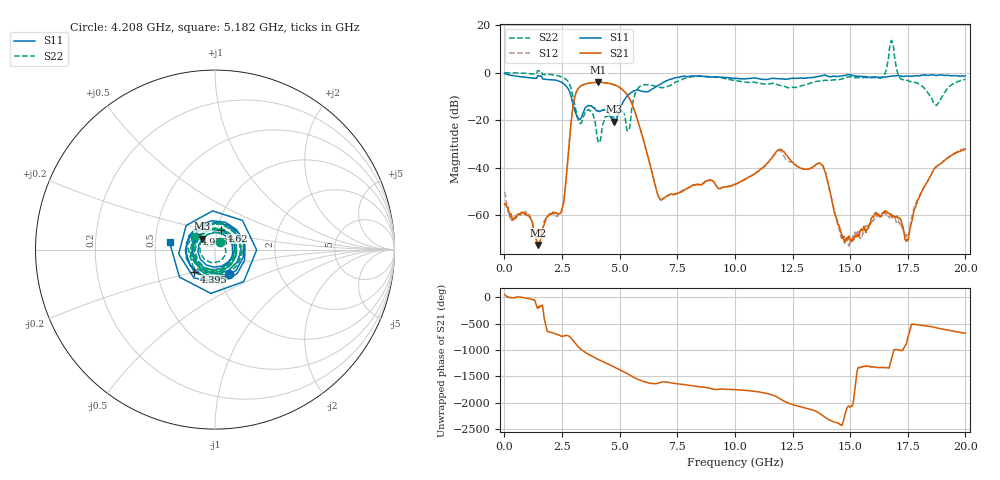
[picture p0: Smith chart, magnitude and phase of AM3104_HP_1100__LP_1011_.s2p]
!Created with skrf (http://scikit-rf.org).
# Hz S RI R 50.0
!freq ReS11 ImS11 ReS21 ImS21 ReS12 ImS12 ReS22 ImS22
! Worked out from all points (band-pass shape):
!   1601 points, 10 MHz to 20 GHz, reference 50 ohm
!   highest |S21| = -4.02 dB at 4.083 GHz (marker M1); lowest = -72.6 dB at 1.459 GHz (marker M2)
!   |S21| within 3 dB of the highest: 3.185 GHz to 5.109 GHz (1.924 GHz wide, 46.4 % of centre)
!   lowest |S11| = -20.6 dB at 4.77 GHz (marker M3), VSWR 1.21, Z = 43.1 + j5.27 ohm
!   |S11| at or under -10 dB: 2.895 GHz to 5.313 GHz (2.417 GHz wide, 58.9 % of centre)
!   |S22| runs from -29.4 to 13.6 dB; largest |S21 - S12| = 0.053
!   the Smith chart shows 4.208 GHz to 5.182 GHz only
!   S11 on the Smith chart (normalised r, x): 4.208 GHz: 1.12, -0.32; 4.395 GHz: 0.77, -0.20; 4.62 GHz: 1.05, +0.23; 4.958 GHz: 0.79, +0.14; 5.182 GHz: 0.59, +0.05
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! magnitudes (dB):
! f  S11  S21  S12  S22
! 10 MHz  -0.4  -55.4  -50.2  -0.1
! 1.459 GHz  -1.3  -72.6  -72.0  0.8
! 2.496 GHz  -4.2  -57.7  -58.1  -1.9
! 2.996 GHz  -14.0  -13.1  -13.1  -10.9
! 3.346 GHz  -18.9  -5.4  -5.5  -21.0
! 4.083 GHz  -16.1  -4.0  -4.1  -29.0
! 4.208 GHz  -16.0  -4.1  -4.1  -26.0
! 4.395 GHz  -15.4  -4.4  -4.4  -18.4
! 4.62 GHz  -19.0  -4.6  -4.8  -18.8
! 4.77 GHz  -20.6  -5.1  -5.2  -19.2
! 4.958 GHz  -17.2  -6.0  -6.0  -17.0
! 5.182 GHz  -11.8  -7.6  -7.7  -17.2
! 6.682 GHz  -5.3  -52.2  -52.2  -6.0
! 10.01 GHz  -2.5  -47.2  -47.3  -3.4
! 11.93 GHz  -2.5  -32.3  -32.7  -5.3
! 13.34 GHz  -2.1  -40.1  -40.1  -4.2
! 13.85 GHz  -1.1  -40.3  -39.9  -3.3
! 14.74 GHz  -1.2  -71.0  -69.6  -2.3
! 16.68 GHz  -1.6  -59.4  -60.8  7.2
! 17.46 GHz  -1.5  -70.2  -68.3  -3.2
! 18.63 GHz  -1.1  -40.9  -41.1  -12.8
! 20 GHz  -1.3  -32.3  -32.0  -2.8
